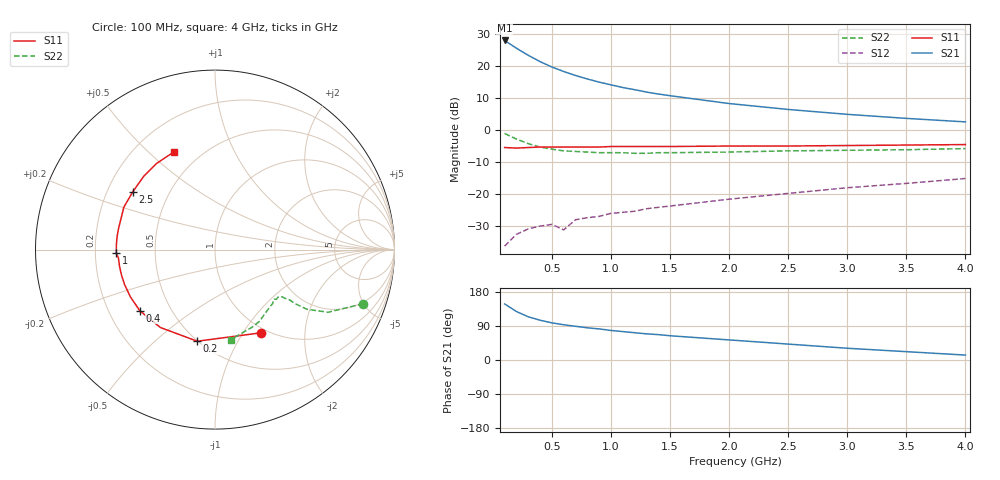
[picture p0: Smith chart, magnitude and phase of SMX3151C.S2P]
! HSMX-3151 Common Emitter
! Vce=10V Ic=15ma
# ghz s ma r 50
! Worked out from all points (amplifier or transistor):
!   20 points, 100 MHz to 4 GHz, reference 50 ohm
!   highest |S21| = 28.1 dB at 100 MHz (marker M1)
!   |S21| within 3 dB of that: start of sweep to 225.4 MHz
!   unconditionally stable (mu >= 1): 573.1 MHz to 649.8 MHz; 848.8 MHz to 3.543 GHz
!   at 400 MHz: K = 0.62, MSG = 25.8 dB, |S12| = -30.2 dB
!   at 1.1 GHz: K = 1.07, MAG = 18.0 dB, |S12| = -25.8 dB
!   at 4 GHz: K = 0.92, MSG = 8.9 dB, |S12| = -15.2 dB
!   S11 on the Smith chart (normalised r, x): 100 MHz: 0.94, -1.21; 200 MHz: 0.50, -0.70; 400 MHz: 0.33, -0.32; 1 GHz: 0.29, -0.02; 2.5 GHz: 0.31, +0.29; 4 GHz: 0.36, +0.60
0.1  0.53 -61.0  25.42 148.0  0.015 64.0  0.88 -20.0
0.2  0.52 -101.0  19.21 128.0  0.023 55.0  0.72 -29.0
0.3  0.53 -125.0  14.86 114.0  0.028 50.0  0.61 -33.0
0.4  0.54 -141.0  11.83 105.0  0.031 50.0  0.54 -34.0
0.5  0.54 -151.0  9.73 98.0  0.033 50.0  0.5 -34.0
0.6  0.54 -159.0  8.28 93.0  0.027 51.0  0.47 -35.0
0.7  0.54 -165.0  7.17 89.0  0.039 52.0  0.46 -35.0
0.8  0.54 -170.0  6.32 85.0  0.042 55.0  0.45 -36.0
0.9  0.54 -175.0  5.64 82.0  0.044 55.0  0.44 -37.0
1  0.55 -178.0  5.11 78.0  0.049 56.0  0.44 -38.0
1.1  0.55 178.0  4.64 75.0  0.051 54.0  0.44 -39.0
1.2  0.55 175.0  4.29 72.0  0.053 58.0  0.43 -40.0
1.3  0.55 172.0  3.94 69.0  0.058 59.0  0.43 -41.0
1.4  0.55 169.0  3.67 67.0  0.061 59.0  0.44 -43.0
1.5  0.55 167.0  3.45 64.0  0.064 61.0  0.44 -44.0
2  0.56 155.0  2.6 53.0  0.082 63.0  0.45 -51.0
2.5  0.56 145.0  2.1 42.0  0.101 63.0  0.47 -58.0
3  0.57 134.0  1.76 31.0  0.124 60.0  0.48 -65.0
3.5  0.58 124.0  1.52 22.0  0.145 59.0  0.49 -73.0
4  0.59 113.0  1.34 13.0  0.173 57.0  0.51 -80.0
